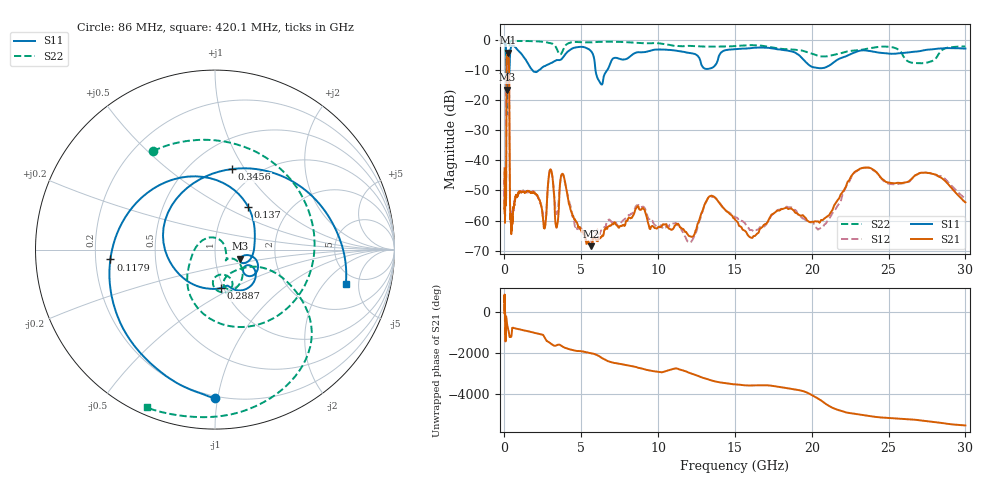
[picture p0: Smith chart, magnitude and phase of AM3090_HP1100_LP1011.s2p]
! Date/Time: Thu, Feb 28, 2019 2:07 PM
! Network Analyzer: Agilent Technologies E8364B Rev: A.07.50.67
! Sweep from 0.010 to 30.000 GHz, 1601 Points, Sweep Type: LOG
! Power Supply: 5.023 V, 0.002 A
# Hz S DB R 50
!freq MagS11 AngS11 MagS21 AngS21 MagS12 AngS12 MagS22 AngS22
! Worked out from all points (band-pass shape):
!   1601 points, 10 MHz to 30 GHz, reference 50 ohm
!   highest |S21| = -4.20 dB at 218.1 MHz (marker M1); lowest = -68.5 dB at 5.612 GHz (marker M2)
!   |S21| within 3 dB of the highest: 143.1 MHz to 288.4 MHz (145.3 MHz wide, 67.3 % of centre)
!   lowest |S11| = -16.5 dB at 168.1 MHz (marker M3), VSWR 1.35, Z = 65.9 - j6.88 ohm
!   |S11| at or under -10 dB: 136 MHz to 324.6 MHz (188.5 MHz wide, 81.9 % of centre); 1.813 GHz to 2.239 GHz (426.1 MHz wide, 21 % of centre); 5.925 GHz to 6.695 GHz (769.5 MHz wide, 12.2 % of centre)
!   |S22| runs from -24.8 to -0.2 dB; largest |S21 - S12| = 0.011
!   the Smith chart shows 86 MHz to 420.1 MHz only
!   S11 on the Smith chart (normalised r, x): 86 MHz: 0.18, -0.98; 117.9 MHz: 0.26, -0.04; 137 MHz: 1.26, +0.66; 288.7 MHz: 0.97, -0.44; 345.6 MHz: 0.77, +0.88; 420.1 MHz: 3.91, -3.48
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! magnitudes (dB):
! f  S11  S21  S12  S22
! 10 MHz  -0.3  -42.7  -45.9  -0.7
! 38.04 MHz  -0.4  -59.2  -55.6  -1.5
! 86 MHz  -1.6  -52.9  -53.6  -3.8
! 117.9 MHz  -4.6  -38.2  -38.3  -5.3
! 137 MHz  -10.4  -10.5  -10.4  -19.3
! 144.7 MHz  -12.9  -6.8  -6.7  -24.8
! 168.1 MHz  -16.5  -4.5  -4.5  -18.9
! 218.1 MHz  -14.3  -4.2  -4.2  -15.3
! 288.7 MHz  -13.3  -7.2  -7.2  -14.8
! 345.6 MHz  -6.8  -49.3  -48.9  -1.1
! 420.1 MHz  -2.5  -60.6  -59.2  -0.4
! 550.5 MHz  -1.9  -58.7  -56.8  -0.3
! 2.084 GHz  -10.6  -51.4  -51.4  -0.5
! 2.623 GHz  -8.7  -62.6  -60.9  -0.7
! 3.017 GHz  -7.7  -43.0  -43.0  -1.1
! 3.402 GHz  -6.7  -62.3  -57.8  -2.9
! 3.798 GHz  -5.9  -44.5  -44.6  -3.5
! 5.612 GHz  -3.6  -68.5  -66.8  -0.8
! 7.926 GHz  -6.3  -60.0  -59.0  -0.7
! 20.41 GHz  -9.3  -60.3  -63.0  -5.3
! 23.48 GHz  -3.5  -42.4  -42.4  -3.0
! 30 GHz  -2.9  -53.9  -52.8  -2.2
